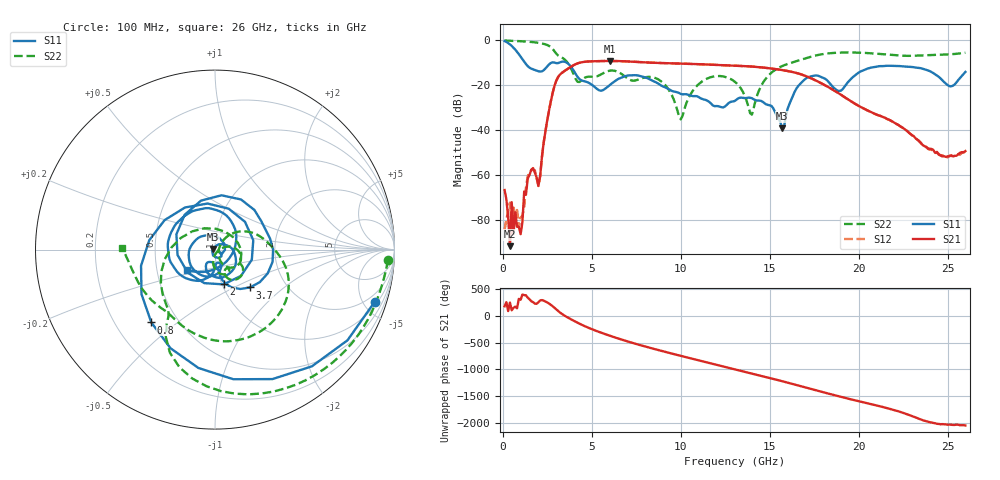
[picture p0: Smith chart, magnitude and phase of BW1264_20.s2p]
!Keysight Technologies,N5245B,MY57181159,A.13.60.06
!Date: Friday, December 18, 2020 23:52:56
!Correction: S11(Full 2 Port(1,2))
!S21(Full 2 Port(1,2))
!S12(Full 2 Port(1,2))
!S22(Full 2 Port(1,2))
!S2P File: Measurements: S11, S21, S12, S22:
# Hz S  dB  R 50
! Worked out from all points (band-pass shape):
!   260 points, 100 MHz to 26 GHz, reference 50 ohm
!   highest |S21| = -9.42 dB at 6 GHz (marker M1); lowest = -91.8 dB at 400 MHz (marker M2)
!   |S21| within 3 dB of the highest: 3.742 GHz to 14.71 GHz (10.97 GHz wide, 119 % of centre)
!   lowest |S11| = -39.3 dB at 15.7 GHz (marker M3), VSWR 1.02, Z = 49 + j0.318 ohm
!   |S11| at or under -10 dB: 1.223 GHz to 3.232 GHz (2.009 GHz wide, 90.2 % of centre); 3.544 GHz to end of sweep
!   |S22| runs from -35.4 to -0.3 dB; largest |S21 - S12| = 0.00049
!   S11 on the Smith chart (normalised r, x): 100 MHz: 1.28, -6.05; 800 MHz: 0.35, -0.41; 2 GHz: 1.02, -0.41; 3.7 GHz: 1.32, -0.61; 26 GHz: 0.71, -0.17
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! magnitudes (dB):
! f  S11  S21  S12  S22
! 100 MHz  -0.6  -66.8  -84.6  -0.3
! 400 MHz  -2.1  -91.8  -72.5  -0.4
! 500 MHz  -2.7  -72.3  -84.1  -0.5
! 800 MHz  -5.4  -83.2  -75.7  -0.6
! 1.1 GHz  -8.6  -81.2  -78.3  -0.7
! 1.2 GHz  -9.8  -67.5  -74.1  -0.7
! 1.6 GHz  -12.8  -57.8  -57.9  -1.0
! 2 GHz  -14.0  -65.0  -65.1  -1.4
! 2.8 GHz  -10.0  -23.7  -23.7  -4.1
! 3.7 GHz  -10.8  -12.6  -12.6  -10.9
! 4.5 GHz  -18.3  -9.9  -9.9  -17.5
! 6 GHz  -20.2  -9.4  -9.4  -13.8
! 8.8 GHz  -19.8  -10.3  -10.3  -17.9
! 10 GHz  -24.1  -10.6  -10.6  -35.4
! 11.2 GHz  -26.3  -10.9  -10.9  -18.5
! 13.1 GHz  -26.8  -11.5  -11.5  -19.1
! 14 GHz  -26.0  -11.9  -11.9  -33.3
! 15.7 GHz  -39.3  -13.5  -13.5  -11.7
! 17.4 GHz  -16.1  -17.4  -17.4  -7.3
! 18.9 GHz  -22.8  -23.9  -23.9  -5.7
! 21.7 GHz  -11.5  -35.5  -35.5  -6.6
! 26 GHz  -14.3  -49.5  -49.7  -5.7
